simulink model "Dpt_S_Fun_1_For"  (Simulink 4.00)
settings: Solver=ode45  SolverMode=SingleTasking  StartTime=0.0  StopTime=0.4  MaxStep=0.001  RelTol=1e-3  AbsTol=1e-3
PreLoadFcn:
  | Load_Param_1
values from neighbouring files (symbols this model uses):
  Cm = 10    [Load_Param_1.m]
  Cw = 10    [Load_Param_1.m]
  Fi = 1    [Load_Param_1.m]
  J = 10    [Load_Param_1.m]
  L = 0.001    [Load_Param_1.m]
  Mnabr = 2500    [Load_Param_1.m]
  R = 0.1    [Load_Param_1.m]
  Tnabr = 0.2    [Load_Param_1.m]
  V = 220    [Load_Param_1.m]

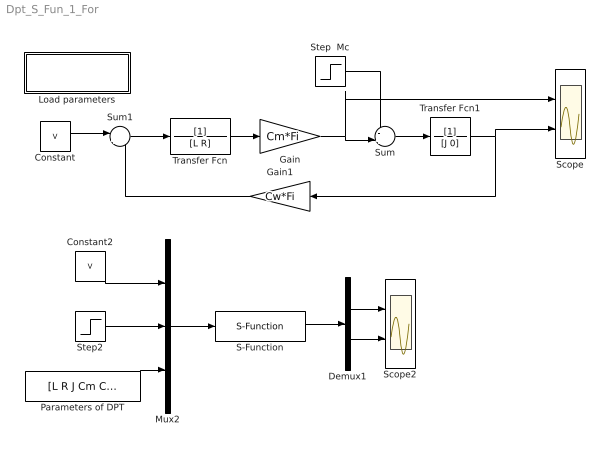
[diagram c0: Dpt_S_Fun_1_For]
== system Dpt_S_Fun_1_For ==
  Constant : Constant  Value=V
  Constant2 : Constant  Value=V
  Demux1 : Demux  Outputs=2  BusSelectionMode=off
  Gain : Gain  Gain=Cm*Fi  Multiplication=Element-wise(K.*u)  SaturateOnIntegerOverflow=on
  Gain1 : Gain  Orientation=left  Gain=Cw*Fi  Multiplication=Element-wise(K.*u)  SaturateOnIntegerOverflow=on
  Load parameters : Subsystem
  Mux2 : Mux  Inputs=3
  Parameters of DPT : Constant  Value=[L R J Cm Cw Fi]
  S-Function : S-Function  FunctionName=DPT_Sfunc_1_For  PortCounts=[]  SFunctionModules=''
  Scope : Scope  NumInputPorts=2
  Scope2 : Scope  NumInputPorts=2
  Step  Mc : Step  Time=Tnabr  Before=0  After=Mnabr  SampleTime=0
  Step2 : Step  Time=Tnabr  Before=0  After=Mnabr  SampleTime=0
  Sum : Sum  Inputs=-+|  SaturateOnIntegerOverflow=on
  Sum1 : Sum  Inputs=|+-  SaturateOnIntegerOverflow=on
  Transfer Fcn : TransferFcn  Numerator=[1]  Denominator=[L R]  AbsoluteTolerance=auto  Realization=auto
  Transfer Fcn1 : TransferFcn  Numerator=[1]  Denominator=[J 0]  AbsoluteTolerance=auto  Realization=auto
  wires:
  Constant/1 -> Sum1/1
  Sum1/1 -> Transfer Fcn/1
  Step  Mc/1 -> Sum/1
  Sum/1 -> Transfer Fcn1/1
  Transfer Fcn/1 -> Gain/1
  Gain/1 -> Sum/2, Scope/1
  Transfer Fcn1/1 -> Gain1/1, Scope/2
  Gain1/1 -> Sum1/2
  S-Function/1 -> Demux1/1
  Demux1/1 -> Scope2/1
  Demux1/2 -> Scope2/2
  Constant2/1 -> Mux2/1
  Step2/1 -> Mux2/2
  Parameters of DPT/1 -> Mux2/3
  Mux2/1 -> S-Function/1

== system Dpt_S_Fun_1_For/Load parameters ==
  note: a
